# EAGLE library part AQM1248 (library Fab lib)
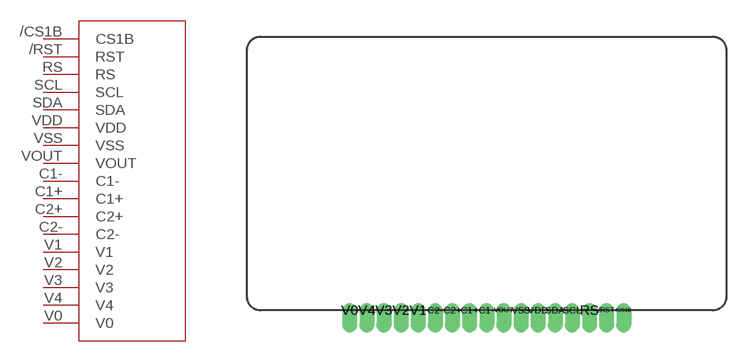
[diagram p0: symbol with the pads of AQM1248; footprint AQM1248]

Designator prefix AQM

## AQM1248  [AQM1248]
/CS1B  CS1B
/RST  RST
C1+  C1+  out
C1-  C1-  out
C2+  C2+  out
C2-  C2-  out
RS  RS
SCL  SCL
SDA  SDA
V0  V0
V1  V1
V2  V2
V3  V3
V4  V4
VDD  VDD  pwr
VOUT  VOUT  out
VSS  VSS  pwr

## Footprint AQM1248 (pad centres in mm)
drill 0.6 pad 0.33 offset: /CS1B 10.16,0; /RST 8.89,0; C1+ -1.27,0; C1- 0,0; C2+ -2.54,0; C2- -3.81,0; RS 7.62,0; SCL 6.35,0; SDA 5.08,0; V0 -10.16,0; V1 -5.08,0; V2 -6.35,0; V3 -7.62,0; V4 -8.89,0; VDD 3.81,0; VOUT 1.27,0; VSS 2.54,0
